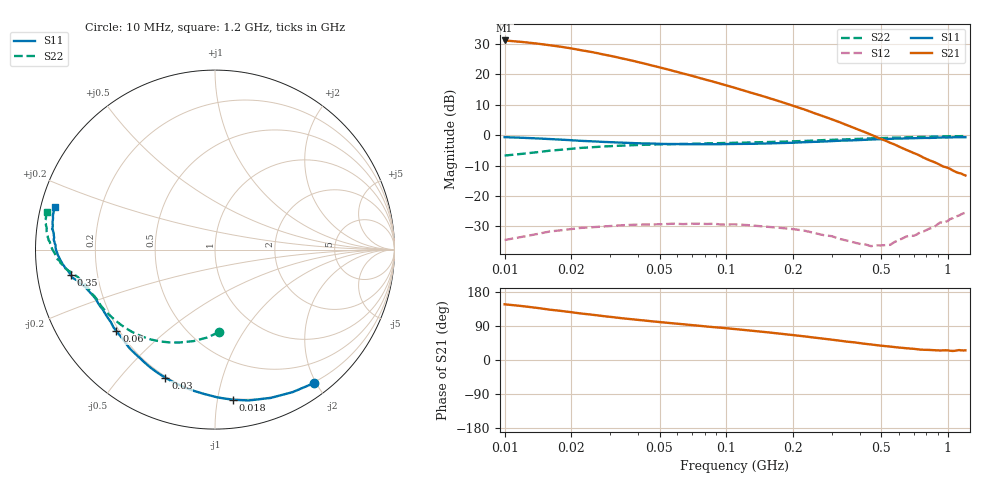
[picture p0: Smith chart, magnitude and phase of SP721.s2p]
!  POLYFET RF DEVICES
!  S PARAMETERS FOR
!  SP721
!  VDS=12.5, IDQ=200MA
# MHZ  S  MA  R  50.0000
! SCATTERING PARAMETERS :
! Freq=MHz Mag[s11] Ang[s11] Mag[s21] Ang[s21] Mag[s12] Ang[s12] Mag[s22] Ang[s22]
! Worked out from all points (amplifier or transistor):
!   95 points, 10 MHz to 1.2 GHz, reference 50 ohm
!   highest |S21| = 31.1 dB at 10 MHz (marker M1)
!   |S21| within 3 dB of that: start of sweep to 21.36 MHz
!   unconditionally stable (mu >= 1): 326.9 MHz to end of sweep
!   at 40 MHz: K = 0.09, MSG = 26.7 dB, |S12| = -29.4 dB
!   at 104 MHz: K = 0.22, MSG = 22.7 dB, |S12| = -29.4 dB
!   at 1.2 GHz: K = 1.15, MAG = 3.8 dB, |S12| = -25.6 dB
!   S11 on the Smith chart (normalised r, x): 10 MHz: 0.19, -1.97; 18 MHz: 0.19, -1.11; 30 MHz: 0.19, -0.67; 60 MHz: 0.19, -0.35; 350 MHz: 0.10, -0.09; 1.2 GHz: 0.04, +0.13
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10  0.9257 -53.5  36.05 147.0  0.01882 57.9  0.4611 -87.4
12  0.9042 -61.4  34.05 142.3  0.02122 52.8  0.4923 -95.3
14  0.8827 -69.4  32.05 137.5  0.02361 47.7  0.5235 -103.2
16  0.8612 -77.4  30.05 132.8  0.02601 42.7  0.5547 -111.0
18  0.8427 -83.2  28.36 129.5  0.02726 39.3  0.5751 -115.9
20  0.8241 -88.9  26.68 126.2  0.0285 35.9  0.5954 -120.7
22  0.8056 -94.6  25 122.8  0.02975 32.5  0.6157 -125.6
24  0.7947 -99.0  23.71 120.5  0.03032 31.0  0.6274 -128.8
28  0.773 -107.8  21.14 115.7  0.03146 27.9  0.6507 -135.1
30  0.7656 -111.2  20.16 113.8  0.03196 26.4  0.658 -137.4
34  0.7508 -117.9  18.18 110.0  0.03295 23.4  0.6724 -141.9
40  0.734 -125.2  15.88 105.9  0.03379 19.1  0.6877 -146.9
50  0.7197 -134.0  13.03 100.2  0.03416 13.6  0.7043 -152.4
60  0.7127 -140.4  10.97 95.8  0.03478 10.5  0.7127 -156.1
82  0.7081 -149.2  8.042 88.2  0.03454 5.0  0.7316 -161.4
110  0.7161 -155.3  5.957 81.5  0.03405 0.1  0.7488 -164.9
125  0.7183 -157.3  5.177 78.3  0.03311 -0.9  0.7557 -166.0
175  0.7398 -161.8  3.569 69.5  0.02981 -5.6  0.7792 -168.6
250  0.7752 -165.9  2.297 59.1  0.02457 -6.1  0.8132 -171.2
350  0.8138 -170.0  1.462 48.5  0.01843 1.4  0.8522 -174.2
550  0.8697 -177.1  0.7464 35.3  0.0157 48.6  0.9045 -179.9
1200  0.9242 165.2  0.2169 25.4  0.05271 83.4  0.9598 167.4
